PROGRAM MAIN
VAR
	{attribute 'OPC.UA.DA':='1'}
	nCounter : INT;
	
	{attribute 'OPC.UA.DA':='1'}
	nNumber : INT;
	
	{attribute 'OPC.UA.DA':='1'}
	fbMathematics : FB_Mathematics;
	
	{attribute 'OPC.UA.DA':='1'}
	iVar1 : INT := 42;
	
	{attribute 'OPC.UA.DA':='1'}
	iVar2 : INT := 43;
	
	{attribute 'OPC.UA.DA':='1'}
	{attribute 'OPC.UA.DA.Access':='1'}
	iVar3_readOnly : INT := 43;	
	
	{attribute 'OPC.UA.DA':='1'}
	{attribute 'OPC.UA.DA.Description' := 'Some description'} 
	iArrayIntVar1 : ARRAY[0..9] OF INT := [10(42)];
	
	{attribute 'OPC.UA.DA':='1'}
	iArrayIntVar2 : ARRAY[0..11] OF INT := [12(41)];	
	
	{attribute 'OPC.UA.DA':='1'}
	{attribute 'OPC.UA.DA.StructuredType':='1'}
	stStructure : ST_Structure;
END_VAR

nCounter := nCounter + 1;

END_PROGRAM
